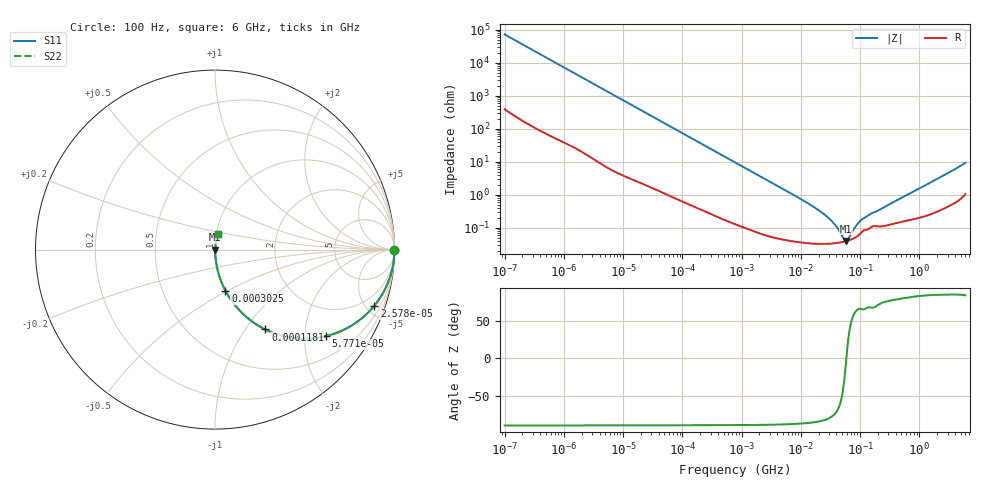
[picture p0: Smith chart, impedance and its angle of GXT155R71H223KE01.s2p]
!Murata Part Number: GXT155R71H223KE01
!These Parameters are Measured in Series Mode Connection
!Data Generated on Jan 08, 2026
!  o--ll--o
!Port1  Port2
!  o------o
!Operation Temp=25[degC], DC Bias Voltage=0[V]
!Freq. Start=100[Hz] Stop=6[GHz] 401[Steps]
# Hz S RI R 50
!Freq.(Hz) S11(Real) S11(Imag) S21(Real) S21(Imag) S12(Real) S12(Imag) S22(Real) S22(Imag)
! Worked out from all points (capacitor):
!   401 points, 100 Hz to 6 GHz, reference 50 ohm
!   read as one part in series: C = 22.2 nF near 109 Hz
!   lowest |Z| = 39.2 mohm at 56.99 MHz (marker M1)
!   series resonance near 58.74 MHz, so ESL is about 330 pH
!   S11 on the Smith chart (normalised r, x): 100 Hz: open; 25.78 kHz: 1.04, -5.66; 57.71 kHz: 1.02, -2.54; 118.1 kHz: 1.01, -1.24; 302.5 kHz: 1.01, -0.49; 6 GHz: 1.02, +0.18
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100  1 -0.00139  9.5e-06 0.00139  9.5e-06 0.00139  1 -0.00139
2008  0.9991 -0.0277  0.000922 0.0277  0.000922 0.0277  0.9991 -0.0277
8416  0.9862 -0.1141  0.0138 0.1141  0.0138 0.1141  0.9862 -0.1141
25777  0.8874 -0.3129  0.1126 0.3129  0.1126 0.3129  0.8874 -0.3129
40335  0.7649 -0.4205  0.2351 0.4205  0.2351 0.4205  0.7649 -0.4205
57709  0.6159 -0.4826  0.3841 0.4826  0.3841 0.4826  0.6159 -0.4826
82567  0.4414 -0.4925  0.5586 0.4925  0.5586 0.4925  0.4414 -0.4925
118133  0.2806 -0.4449  0.7194 0.4449  0.7194 0.4449  0.2806 -0.4449
184852  0.1394 -0.3415  0.8606 0.3415  0.8606 0.3415  0.1394 -0.3415
302498  0.0584 -0.2293  0.9416 0.2293  0.9416 0.2293  0.0584 -0.2293
774597  0.0104 -0.0948  0.9896 0.0948  0.9896 0.0948  0.0104 -0.0948
2481164  0.0015 -0.0301  0.9985 0.0301  0.9985 0.0301  0.0015 -0.0301
1.555665e7  0.000349 -0.00453  0.9997 0.00453  0.9997 0.00453  0.000349 -0.00453
3.330331e7  0.000331 -0.00155  0.9997 0.00155  0.9997 0.00155  0.000331 -0.00155
4.165952e7  0.000344 -0.000905  0.9997 0.000905  0.9997 0.000905  0.000344 -0.000905
5.211241e7  0.00037 -0.000309  0.9996 0.000309  0.9996 0.000309  0.00037 -0.000309
5.699437e7  0.000385 -7.76e-05  0.9996 7.76e-05  0.9996 7.76e-05  0.000385 -7.76e-05
6.233367e7  0.000403 0.000154  0.9996 -0.000154  0.9996 -0.000154  0.000403 0.000154
8.527865e7  0.000516 0.000989  0.9995 -0.000989  0.9995 -0.000989  0.000516 0.000989
1.066761e8  0.000741 0.0016  0.9993 -0.0016  0.9993 -0.0016  0.000741 0.0016
3.124326e8  0.00124 0.00496  0.9988 -0.00496  0.9988 -0.00496  0.00124 0.00496
6e9  0.0185 0.0895  0.9815 -0.0895  0.9815 -0.0895  0.0185 0.0895
